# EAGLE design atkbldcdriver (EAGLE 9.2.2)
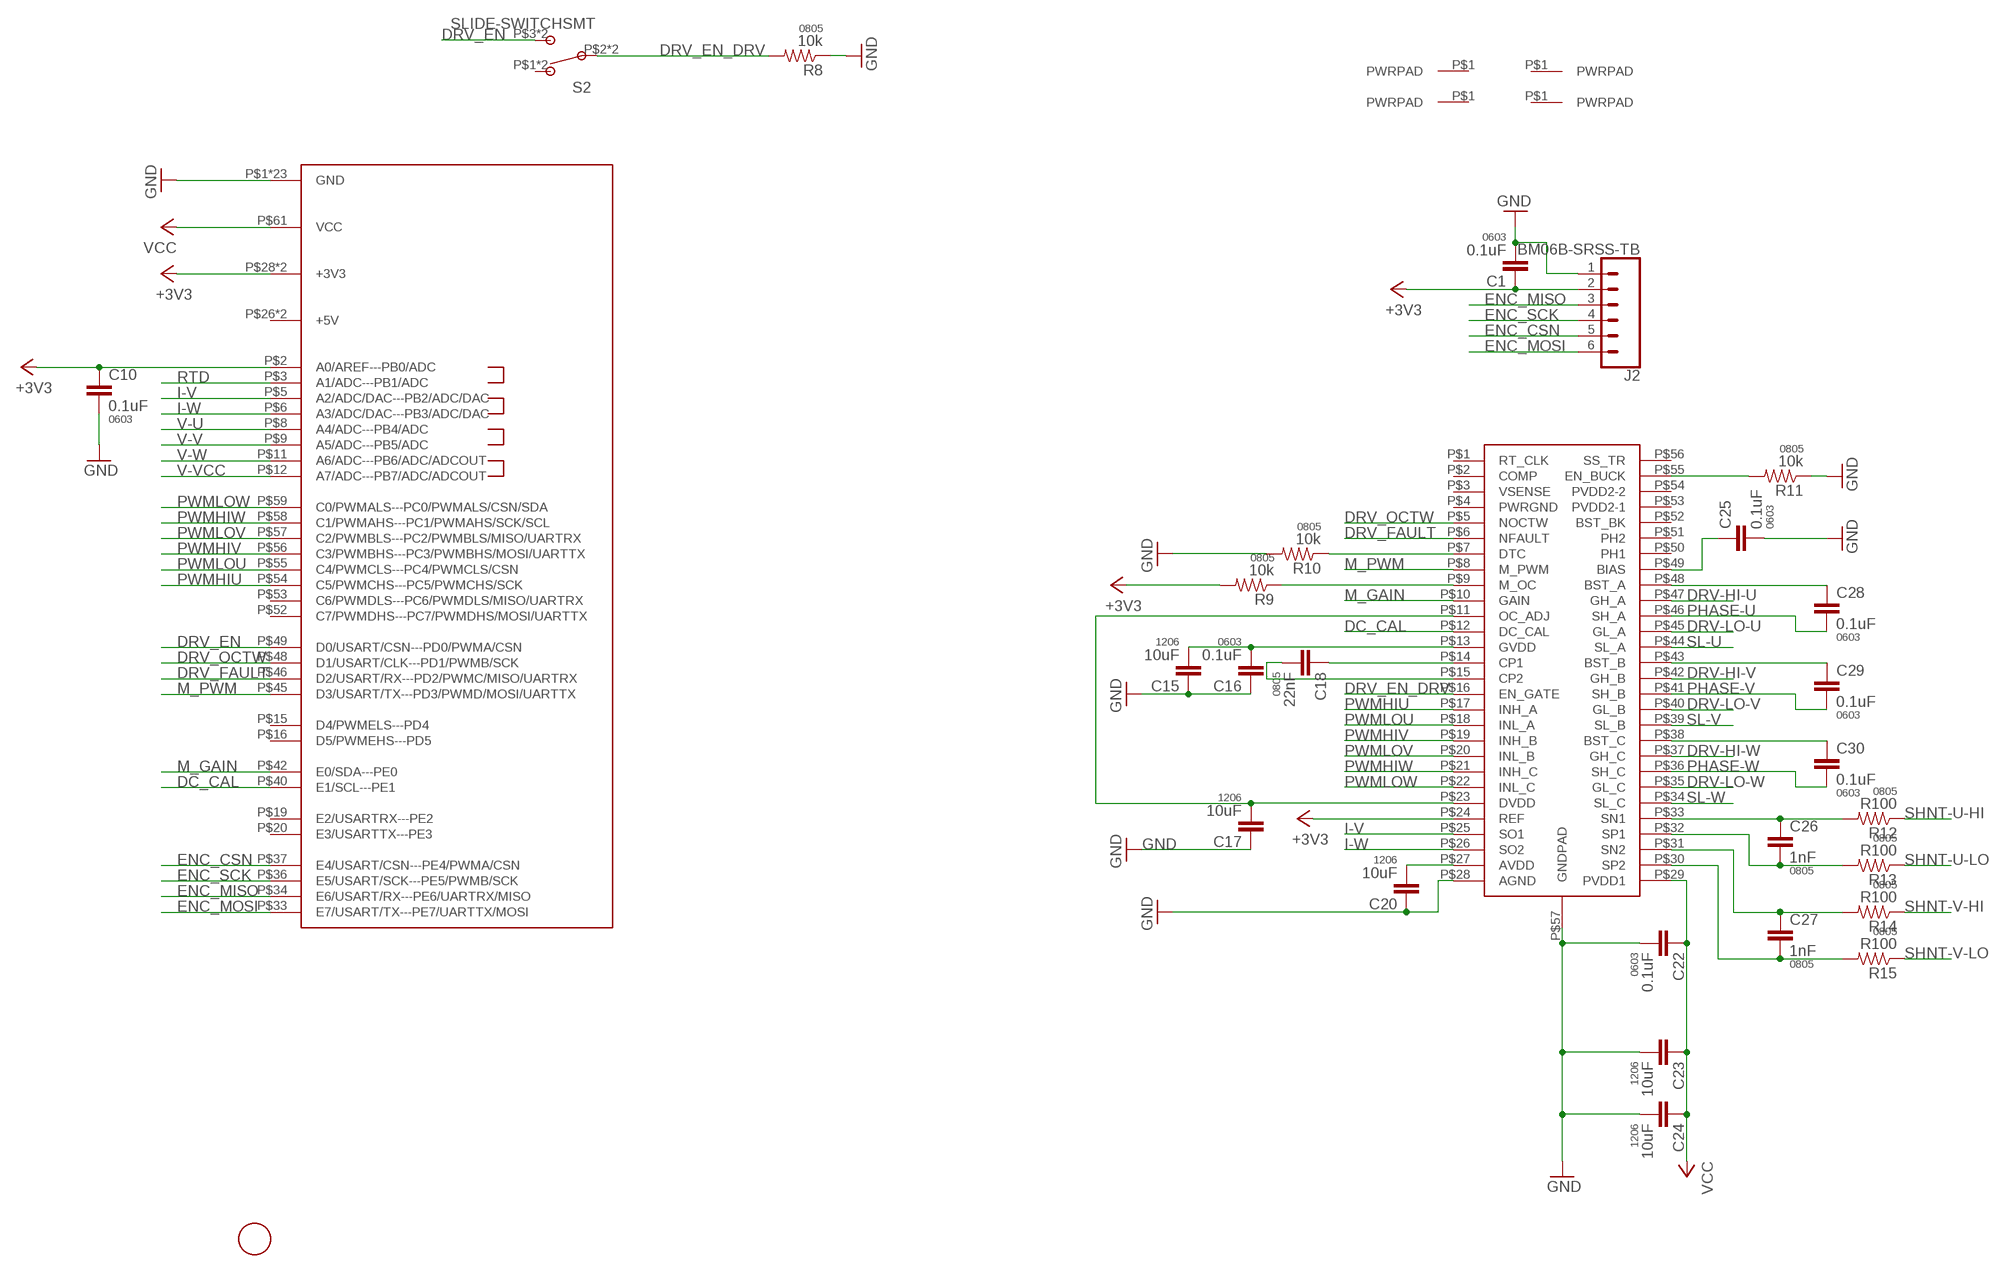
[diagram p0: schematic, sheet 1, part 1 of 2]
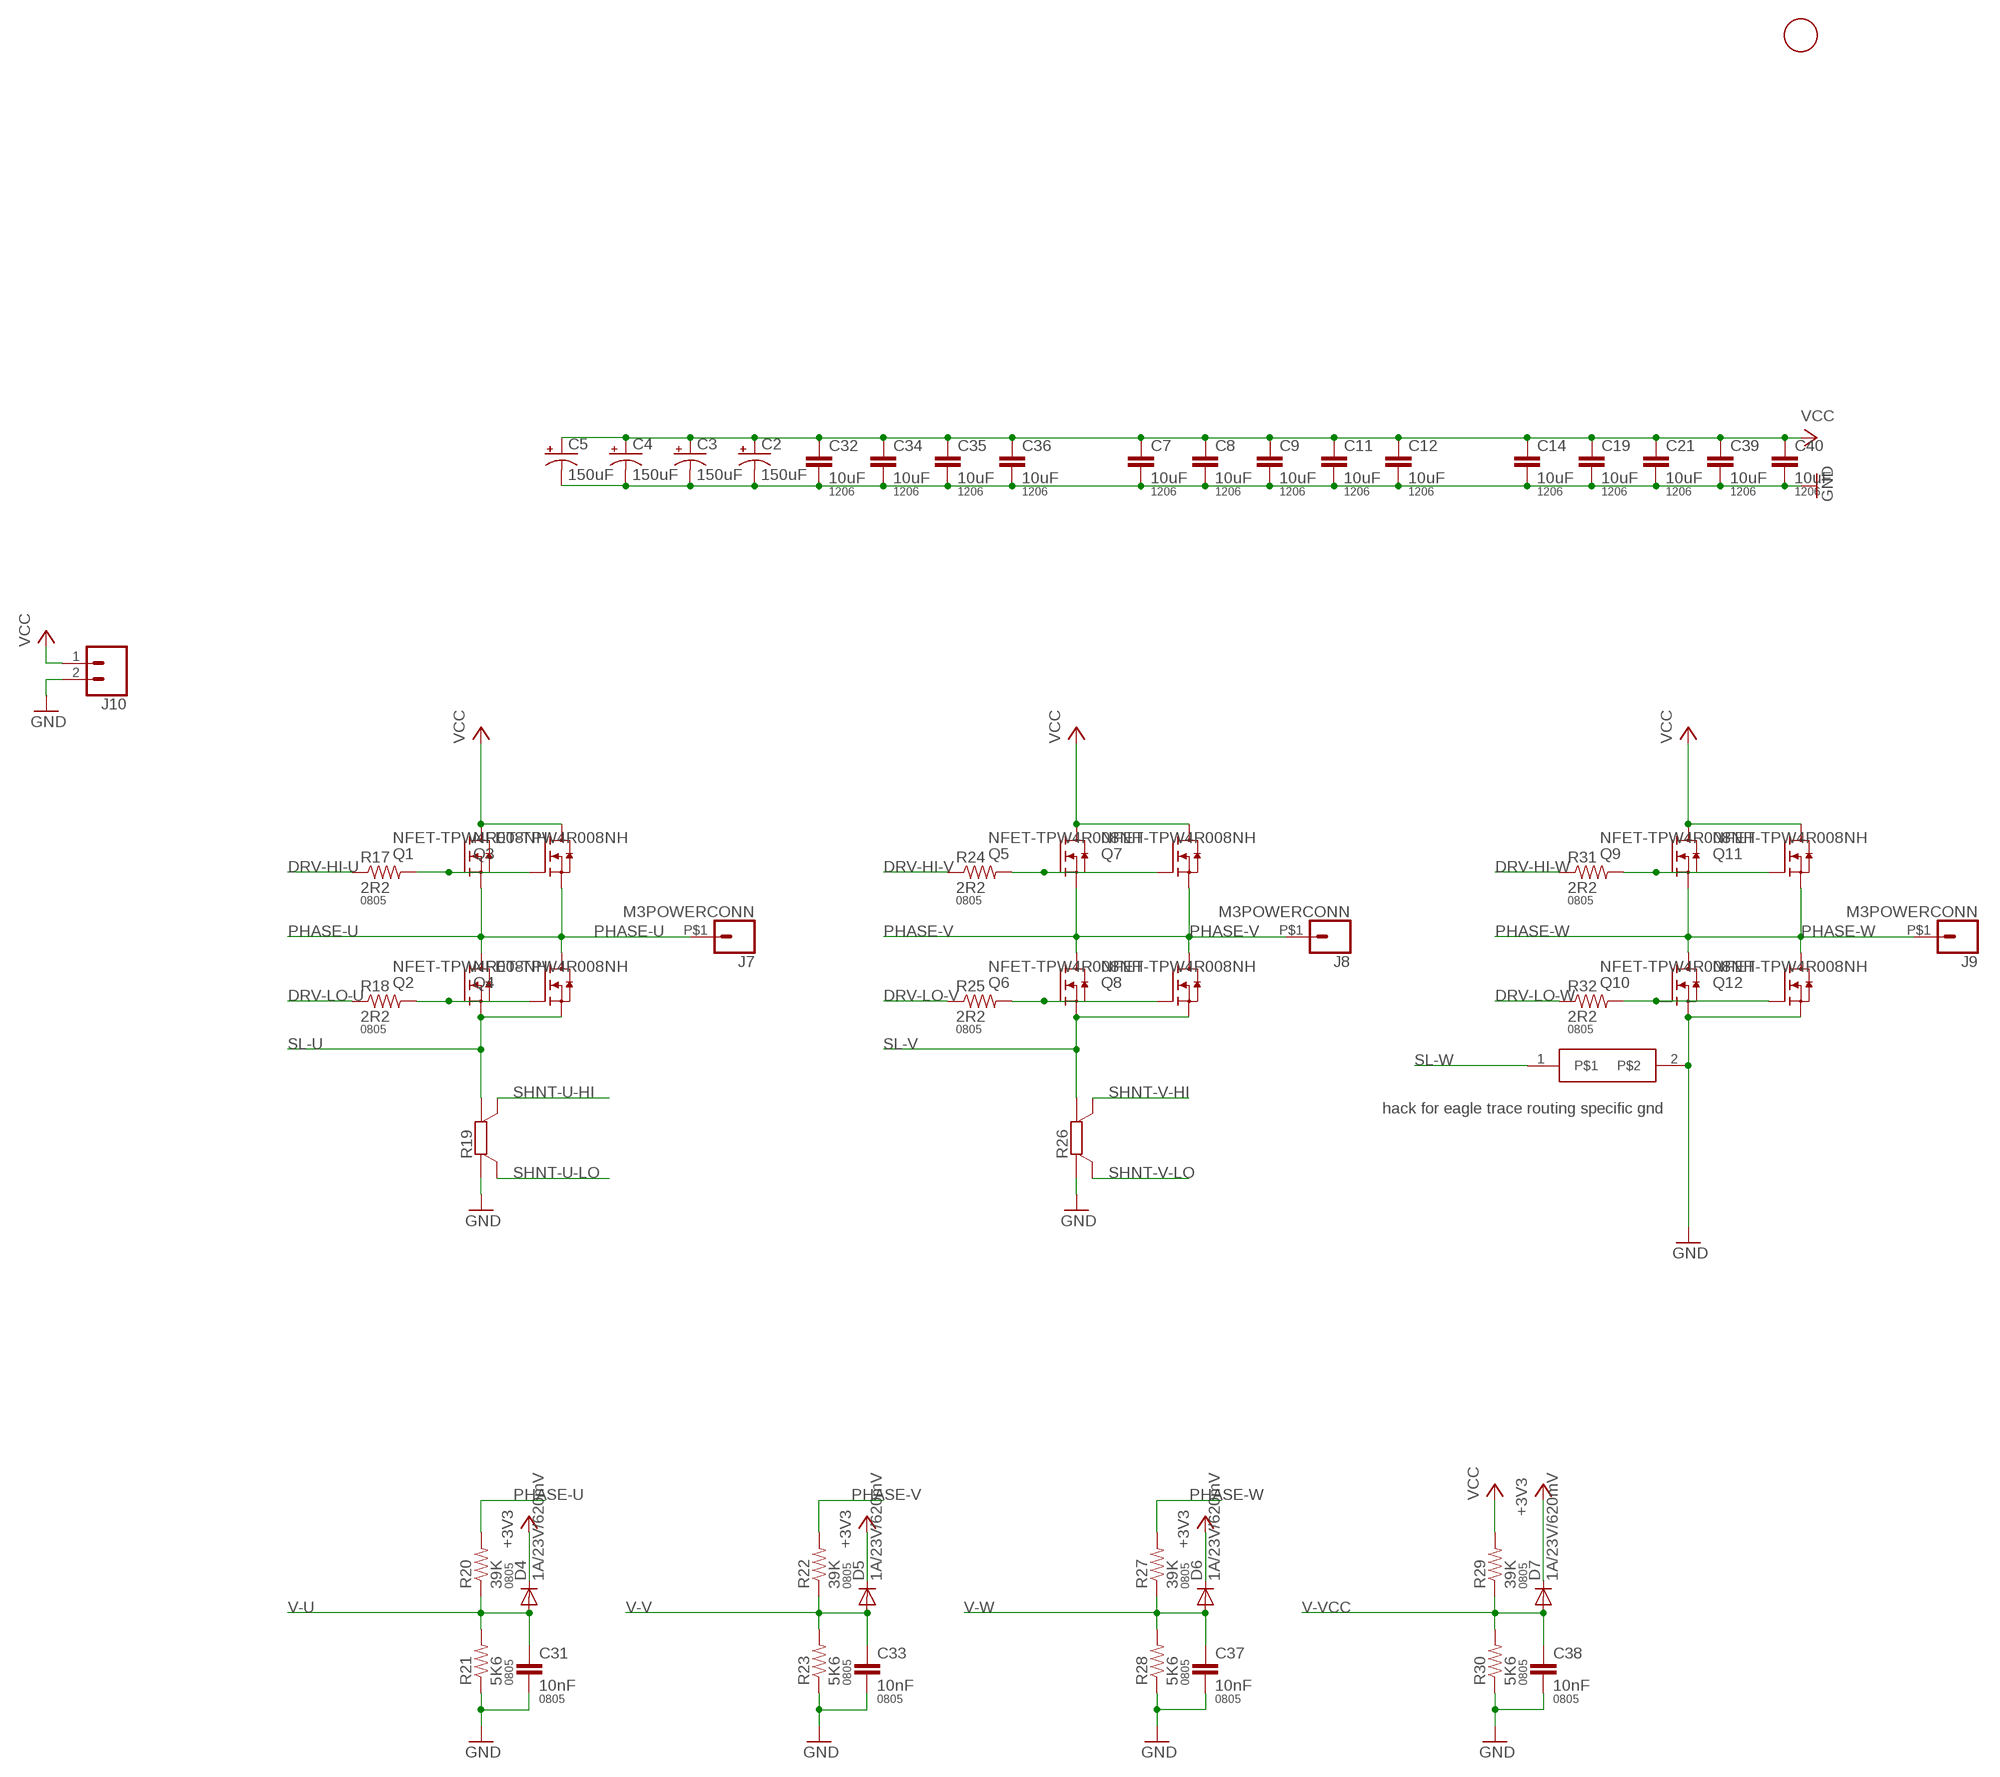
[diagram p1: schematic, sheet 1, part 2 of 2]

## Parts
C1  0.1uF  CAP0603-CAP  [0603-CAP]
C2  150uF  CAP-POL-6.6X6.6  [6.6X6.6-CAP]
C3  150uF  CAP-POL-6.6X6.6  [6.6X6.6-CAP]
C4  150uF  CAP-POL-6.6X6.6  [6.6X6.6-CAP]
C5  150uF  CAP-POL-6.6X6.6  [6.6X6.6-CAP]
C7  10uF  CAP1206  [1206]
C8  10uF  CAP1206  [1206]
C9  10uF  CAP1206  [1206]
C10  0.1uF  CAP0603-CAP  [0603-CAP]
C11  10uF  CAP1206  [1206]
C12  10uF  CAP1206  [1206]
C14  10uF  CAP1206  [1206]
C15  10uF  CAP1206  [1206]
C16  0.1uF  CAP0603-CAP  [0603-CAP]
C17  10uF  CAP1206  [1206]
C18  22nF  CAP0805  [0805]
C19  10uF  CAP1206  [1206]
C20  10uF  CAP1206  [1206]
C21  10uF  CAP1206  [1206]
C22  0.1uF  CAP0603-CAP  [0603-CAP]
C23  10uF  CAP1206  [1206]
C24  10uF  CAP1206  [1206]
C25  0.1uF  CAP0603-CAP  [0603-CAP]
C26  1nF  CAP0805  [0805]
C27  1nF  CAP0805  [0805]
C28  0.1uF  CAP0603-CAP  [0603-CAP]
C29  0.1uF  CAP0603-CAP  [0603-CAP]
C30  0.1uF  CAP0603-CAP  [0603-CAP]
C31  10nF  CAP0805  [0805]
C32  10uF  CAP1206  [1206]
C33  10nF  CAP0805  [0805]
C34  10uF  CAP1206  [1206]
C35  10uF  CAP1206  [1206]
C36  10uF  CAP1206  [1206]
C37  10nF  CAP0805  [0805]
C38  10nF  CAP0805  [0805]
C39  10uF  CAP1206  [1206]
C40  10uF  CAP1206  [1206]
D4  1A/23V/620mV  DIODEDIODE  [0805-DIODE]
D5  1A/23V/620mV  DIODEDIODE  [0805-DIODE]
D6  1A/23V/620mV  DIODEDIODE  [0805-DIODE]
D7  1A/23V/620mV  DIODEDIODE  [0805-DIODE]
J1  FIDUCIALRCT  [FIDUCIAL_RECT_1MM]
J2  BM06B-SRSS-TB  JST_6_PIN_HORIZONTAL  [JST-6-SMD-HORI-1.0MM]
J3  PWRPADM3  [PWRPAD_3-25MM]
J4  PWRPADM3  [PWRPAD_3-25MM]
J5  PWRPADM3  [PWRPAD_3-25MM]
J6  PWRPADM3  [PWRPAD_3-25MM]
J7  M3POWERCONN  [M3POWERCONN]
J8  M3POWERCONN  [M3POWERCONN]
J9  M3POWERCONN  [M3POWERCONN]
J10  CONN_021X02_NO_SILK  [1X02_NO_SILK]
J21  SL-LINK  [SL-LINK]
J22  FIDUCIALRCT  [FIDUCIAL_RECT_1MM]
J24  ATK-BFPPFX8-DAUGHTER  [ATK-BFPP-TOP-FX8-60]
Q1  NFET-TPW4R008NH  [DSOP-ADVANCE]
Q2  NFET-TPW4R008NH  [DSOP-ADVANCE]
Q3  NFET-TPW4R008NH  [DSOP-ADVANCE]
Q4  NFET-TPW4R008NH  [DSOP-ADVANCE]
Q5  NFET-TPW4R008NH  [DSOP-ADVANCE]
Q6  NFET-TPW4R008NH  [DSOP-ADVANCE]
Q7  NFET-TPW4R008NH  [DSOP-ADVANCE]
Q8  NFET-TPW4R008NH  [DSOP-ADVANCE]
Q9  NFET-TPW4R008NH  [DSOP-ADVANCE]
Q10  NFET-TPW4R008NH  [DSOP-ADVANCE]
Q11  NFET-TPW4R008NH  [DSOP-ADVANCE]
Q12  NFET-TPW4R008NH  [DSOP-ADVANCE]
R8  10k  RESISTOR0805-RES  [0805]
R9  10k  RESISTOR0805-RES  [0805]
R10  10k  RESISTOR0805-RES  [0805]
R11  10k  RESISTOR0805-RES  [0805]
R12  R100  RESISTOR0805-RES  [0805]
R13  R100  RESISTOR0805-RES  [0805]
R14  R100  RESISTOR0805-RES  [0805]
R15  R100  RESISTOR0805-RES  [0805]
R17  2R2  RESISTOR0805-RES  [0805]
R18  2R2  RESISTOR0805-RES  [0805]
R19  R_SHUNT2512  [R2512]
R20  39K  RESISTOR0805-RES  [0805]
R21  5K6  RESISTOR0805-RES  [0805]
R22  39K  RESISTOR0805-RES  [0805]
R23  5K6  RESISTOR0805-RES  [0805]
R24  2R2  RESISTOR0805-RES  [0805]
R25  2R2  RESISTOR0805-RES  [0805]
R26  R_SHUNT2512  [R2512]
R27  39K  RESISTOR0805-RES  [0805]
R28  5K6  RESISTOR0805-RES  [0805]
R29  39K  RESISTOR0805-RES  [0805]
R30  5K6  RESISTOR0805-RES  [0805]
R31  2R2  RESISTOR0805-RES  [0805]
R32  2R2  RESISTOR0805-RES  [0805]
S2  SLIDE-SWITCHSMT  [SLIDESWITCH-CL-SB-22A]
U5  DRV8302  [HTSSOP-56]

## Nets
+3V3: C1.1 C10.1 D4.2(C) D5.2(C) D6.2(C) D7.2(C) J2.2 J24.P$2(A0/AREF---PB0/ADC) J24.P$28(+3V3) J24.P$29(+3V3) R9.2 U5.P$24(REF)
CP1: C18.1 U5.P$14(CP1)
CP2: C18.2 U5.P$15(CP2)
DC_CAL: J24.P$40(E1/SCL---PE1) U5.P$12(DC_CAL)
DRV-HI-U: R17.1 U5.P$47(GH_A)
DRV-HI-V: R24.1 U5.P$42(GH_B)
DRV-HI-W: R31.1 U5.P$37(GH_C)
DRV-LO-U: R18.1 U5.P$45(GL_A)
DRV-LO-V: R25.1 U5.P$40(GL_B)
DRV-LO-W: R32.1 U5.P$35(GL_C)
DRV_EN: J24.P$49(D0/USART/CSN---PD0/PWMA/CSN) S2.P$3 S2.P$6
DRV_EN_DRV: R8.2 S2.P$2 S2.P$5 U5.P$16(EN_GATE)
DRV_FAULT: J24.P$46(D2/USART/RX---PD2/PWMC/MISO/UARTRX) U5.P$6(NFAULT)
DRV_OCTW: J24.P$48(D1/USART/CLK---PD1/PWMB/SCK) U5.P$5(NOCTW)
ENC_CSN: J2.5 J24.P$37(E4/USART/CSN---PE4/PWMA/CSN)
ENC_MISO: J2.3 J24.P$34(E6/USART/RX---PE6/UARTRX/MISO)
ENC_MOSI: J2.6 J24.P$33(E7/USART/TX---PE7/UARTTX/MOSI)
ENC_SCK: J2.4 J24.P$36(E5/USART/SCK---PE5/PWMB/SCK)
GND: C1.2 C2.- C3.- C4.- C5.- C7.2 C8.2 C9.2 C10.2 C11.2 C12.2 C14.2 C15.1 C16.1 C17.1 C19.2 C20.1 C21.2 C22.2 C23.2 C24.2 C25.2 C31.2 C32.2 C33.2 C34.2 C35.2 C36.2 C37.2 C38.2 C39.2 C40.2 J2.1 J10.2 J21.2 J24.P$1(GND) J24.P$4(GND) J24.P$7(GND) J24.P$10(GND) J24.P$13(GND) J24.P$14(GND) J24.P$17(GND) J24.P$18(GND) J24.P$21(GND) J24.P$30(GND) J24.P$31(GND) J24.P$32(GND) J24.P$35(GND) J24.P$38(GND) J24.P$39(GND) J24.P$41(GND) J24.P$43(GND) J24.P$44(GND) J24.P$47(GND) J24.P$50(GND) J24.P$51(GND) J24.P$60(GND) J24.P$62(GND) Q10.P$1(S) Q10.P$2(S) Q10.P$3(S) Q12.P$1(S) Q12.P$2(S) Q12.P$3(S) R8.1 R10.2 R11.1 R19.B R21.1 R23.1 R26.B R28.1 R30.1 U5.P$28(AGND) U5.P$57(GNDPAD)
I-V: J24.P$5(A2/ADC/DAC---PB2/ADC/DAC) U5.P$25(SO1)
I-W: J24.P$6(A3/ADC/DAC---PB3/ADC/DAC) U5.P$26(SO2)
M_GAIN: J24.P$42(E0/SDA---PE0) U5.P$10(GAIN)
M_PWM: J24.P$45(D3/USART/TX---PD3/PWMD/MOSI/UARTTX) U5.P$8(M_PWM)
N$2: Q2.P$4(G) Q4.P$4(G) R18.2
N$3: Q1.P$4(G) Q3.P$4(G) R17.2
N$4: Q5.P$4(G) Q7.P$4(G) R24.2
N$5: Q9.P$4(G) Q11.P$4(G) R31.2
N$6: Q10.P$4(G) Q12.P$4(G) R32.2
N$7: C30.1 U5.P$38(BST_C)
N$8: C29.1 U5.P$43(BST_B)
N$9: C28.1 U5.P$48(BST_A)
N$10: R11.2 U5.P$55(EN_BUCK)
N$11: C20.2 U5.P$27(AVDD)
N$13: C26.1 R12.2 U5.P$33(SN1)
N$14: C26.2 R13.2 U5.P$32(SP1)
N$15: C27.1 R14.2 U5.P$31(SN2)
N$16: C27.2 R15.2 U5.P$30(SP2)
N$18: C15.2 C16.2 U5.P$13(GVDD)
N$19: C25.1 U5.P$49(BIAS)
N$20: C17.2 U5.P$11(OC_ADJ) U5.P$23(DVDD)
N$21: R10.1 U5.P$7(DTC)
N$24: Q6.P$4(G) Q8.P$4(G) R25.2
N$25: R9.1 U5.P$9(M_OC)
PHASE-U: C28.2 J7.P$1 Q1.P$1(S) Q1.P$2(S) Q1.P$3(S) Q2.P$5(D) Q3.P$1(S) Q3.P$2(S) Q3.P$3(S) Q4.P$5(D) R20.2 U5.P$46(SH_A)
PHASE-V: C29.2 J8.P$1 Q5.P$1(S) Q5.P$2(S) Q5.P$3(S) Q6.P$5(D) Q7.P$1(S) Q7.P$2(S) Q7.P$3(S) Q8.P$5(D) R22.2 U5.P$41(SH_B)
PHASE-W: C30.2 J9.P$1 Q9.P$1(S) Q9.P$2(S) Q9.P$3(S) Q10.P$5(D) Q11.P$1(S) Q11.P$2(S) Q11.P$3(S) Q12.P$5(D) R27.2 U5.P$36(SH_C)
PWMHIU: J24.P$54(C5/PWMCHS---PC5/PWMCHS/SCK) U5.P$17(INH_A)
PWMHIV: J24.P$56(C3/PWMBHS---PC3/PWMBHS/MOSI/UARTTX) U5.P$19(INH_B)
PWMHIW: J24.P$58(C1/PWMAHS---PC1/PWMAHS/SCK/SCL) U5.P$21(INH_C)
PWMLOU: J24.P$55(C4/PWMCLS---PC4/PWMCLS/CSN) U5.P$18(INL_A)
PWMLOV: J24.P$57(C2/PWMBLS---PC2/PWMBLS/MISO/UARTRX) U5.P$20(INL_B)
PWMLOW: J24.P$59(C0/PWMALS---PC0/PWMALS/CSN/SDA) U5.P$22(INL_C)
RTD: J24.P$3(A1/ADC---PB1/ADC)
SHNT-U-HI: R12.1 R19.SA
SHNT-U-LO: R13.1 R19.SB
SHNT-V-HI: R14.1 R26.SA
SHNT-V-LO: R15.1 R26.SB
SL-U: Q2.P$1(S) Q2.P$2(S) Q2.P$3(S) Q4.P$1(S) Q4.P$2(S) Q4.P$3(S) R19.A U5.P$44(SL_A)
SL-V: Q6.P$1(S) Q6.P$2(S) Q6.P$3(S) Q8.P$1(S) Q8.P$2(S) Q8.P$3(S) R26.A U5.P$39(SL_B)
SL-W: J21.1 U5.P$34(SL_C)
V-U: C31.1 D4.1(A) J24.P$8(A4/ADC---PB4/ADC) R20.1 R21.2
V-V: C33.1 D5.1(A) J24.P$9(A5/ADC---PB5/ADC) R22.1 R23.2
V-VCC: C38.1 D7.1(A) J24.P$12(A7/ADC---PB7/ADC/ADCOUT) R29.1 R30.2
V-W: C37.1 D6.1(A) J24.P$11(A6/ADC---PB6/ADC/ADCOUT) R27.1 R28.2
VCC: C2.+ C3.+ C4.+ C5.+ C7.1 C8.1 C9.1 C11.1 C12.1 C14.1 C19.1 C21.1 C22.1 C23.1 C24.1 C32.1 C34.1 C35.1 C36.1 C39.1 C40.1 J10.1 J24.P$61(VCC) Q1.P$5(D) Q3.P$5(D) Q5.P$5(D) Q7.P$5(D) Q9.P$5(D) Q11.P$5(D) R29.2 U5.P$29(PVDD1)
Unconnected: J3.P$1(PWRPAD) J4.P$1(PWRPAD) J5.P$1(PWRPAD) J6.P$1(PWRPAD) J24.P$15(D4/PWMELS---PD4) J24.P$16(D5/PWMEHS---PD5) J24.P$19(E2/USARTRX---PE2) J24.P$20(E3/USARTTX---PE3) J24.P$26(+5V) J24.P$27(+5V) J24.P$52(C7/PWMDHS---PC7/PWMDHS/MOSI/UARTTX) J24.P$53(C6/PWMDLS---PC6/PWMDLS/MISO/UARTRX) S2.P$1 S2.P$4 U5.P$1(RT_CLK) U5.P$2(COMP) U5.P$3(VSENSE) U5.P$4(PWRGND) U5.P$50(PH1) U5.P$51(PH2) U5.P$52(BST_BK) U5.P$53(PVDD2-1) U5.P$54(PVDD2-2) U5.P$56(SS_TR)

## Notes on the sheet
- hack for eagle trace routing specific gnd

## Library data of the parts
C1 C10 C16 C22 C25 C28-C30 = borkedlabs-passives:CAP: Capacitor; PACKAGE: 0603
C2-C5 = borkedlabs-passives:CAP-POL
C7-C9 C11 C12 C14 C15 C17 C19-C21 C23 C24 C32 C34-C36 C39 C40 = borkedlabs-passives:CAP: Capacitor; PACKAGE: 1206
C18 C26 C27 C31 C33 C37 C38 = borkedlabs-passives:CAP: Capacitor; PACKAGE: 0805
D4-D7 = passives:DIODE: DIODE
J1 J22 = connector:FIDUCIAL: For use by pick and place machines to calibrate the vision/machine, 1mm
J2 = connector:JST_6_PIN_HORIZONTAL: JST 6 pin horizontal connector JST-SH type. Here is the connector we sell at SparkFun: name (XXX-00000) Datasheet It was used on these SparkFun products: name (XXX-00000) name (XXX-00000); PROD_ID: XXX-00000
J3-J6 = power:PWRPAD
J7-J9 = connector:M3POWERCONN
J10 = SparkFun-Connectors:CONN_02: Multi connection point. Often used as Generic Header-pin footprint for 0.1 inch spaced/style header connections
J21 = power:SL-LINK
J24 = connector:ATK-BFPP
Q1-Q12 = power:NFET-TPW4R008NH
R8-R15 R17 R18 R20-R25 R27-R32 = borkedlabs-passives:RESISTOR: Resistor; PACKAGE: 0805
R19 R26 = power:R_SHUNT: Resistor Basic schematic elements and footprints for 0603, 1206, and PTH resistors.
S2 = fab:SLIDE-SWITCH: SMD slide-switch AYZ0102AGRLC as found in the fablab inventory. Includes the mounting holes. Made by Zaerc.
U5 = power:DRV8302

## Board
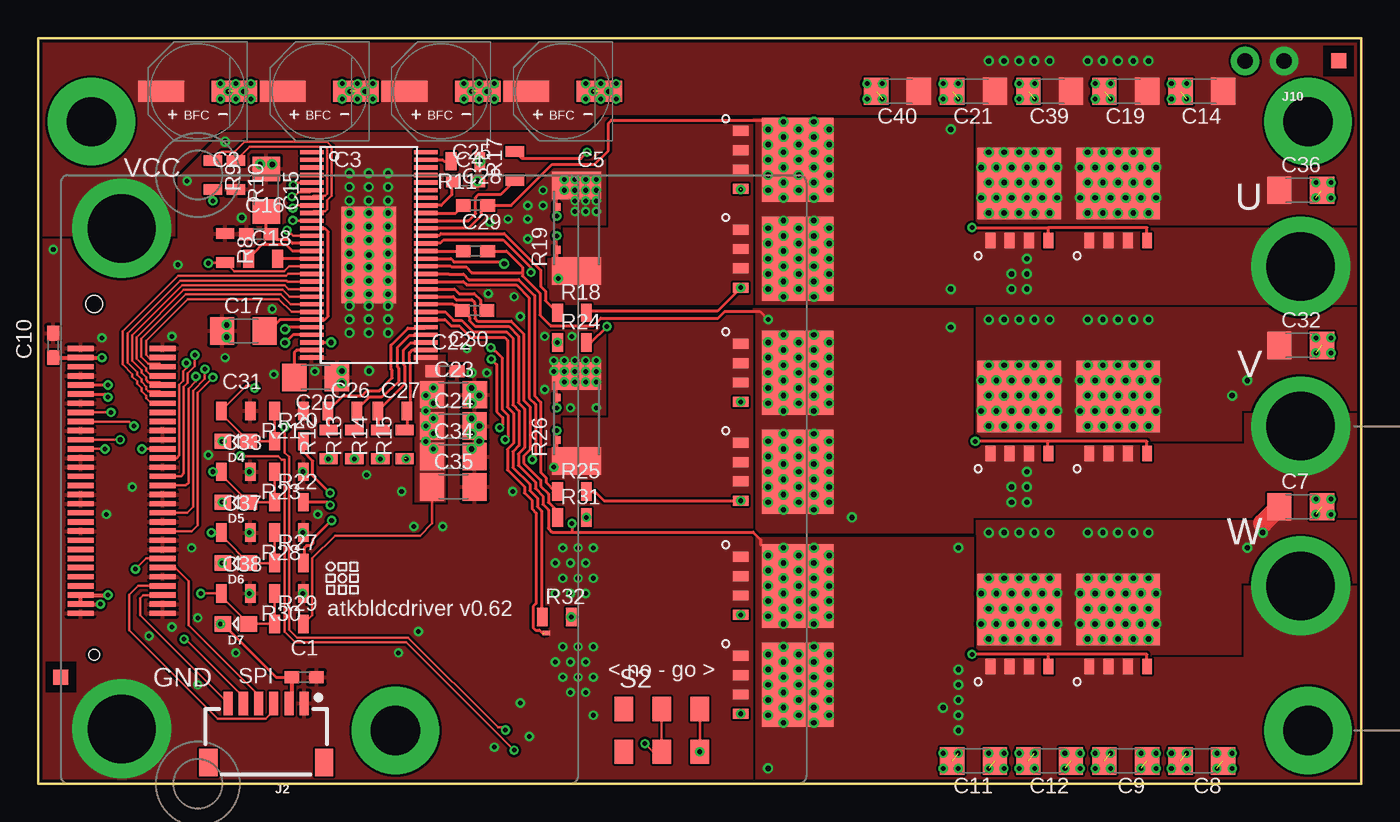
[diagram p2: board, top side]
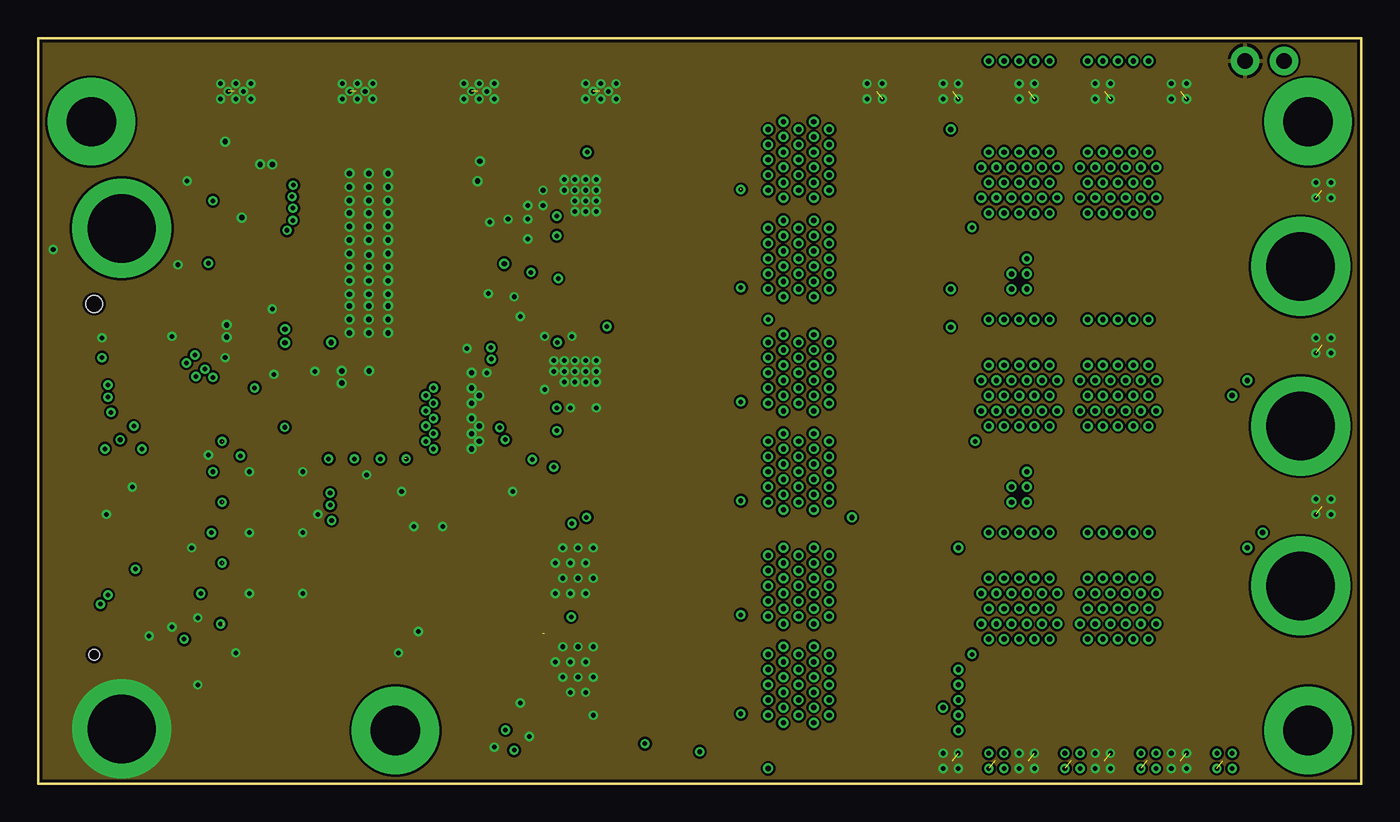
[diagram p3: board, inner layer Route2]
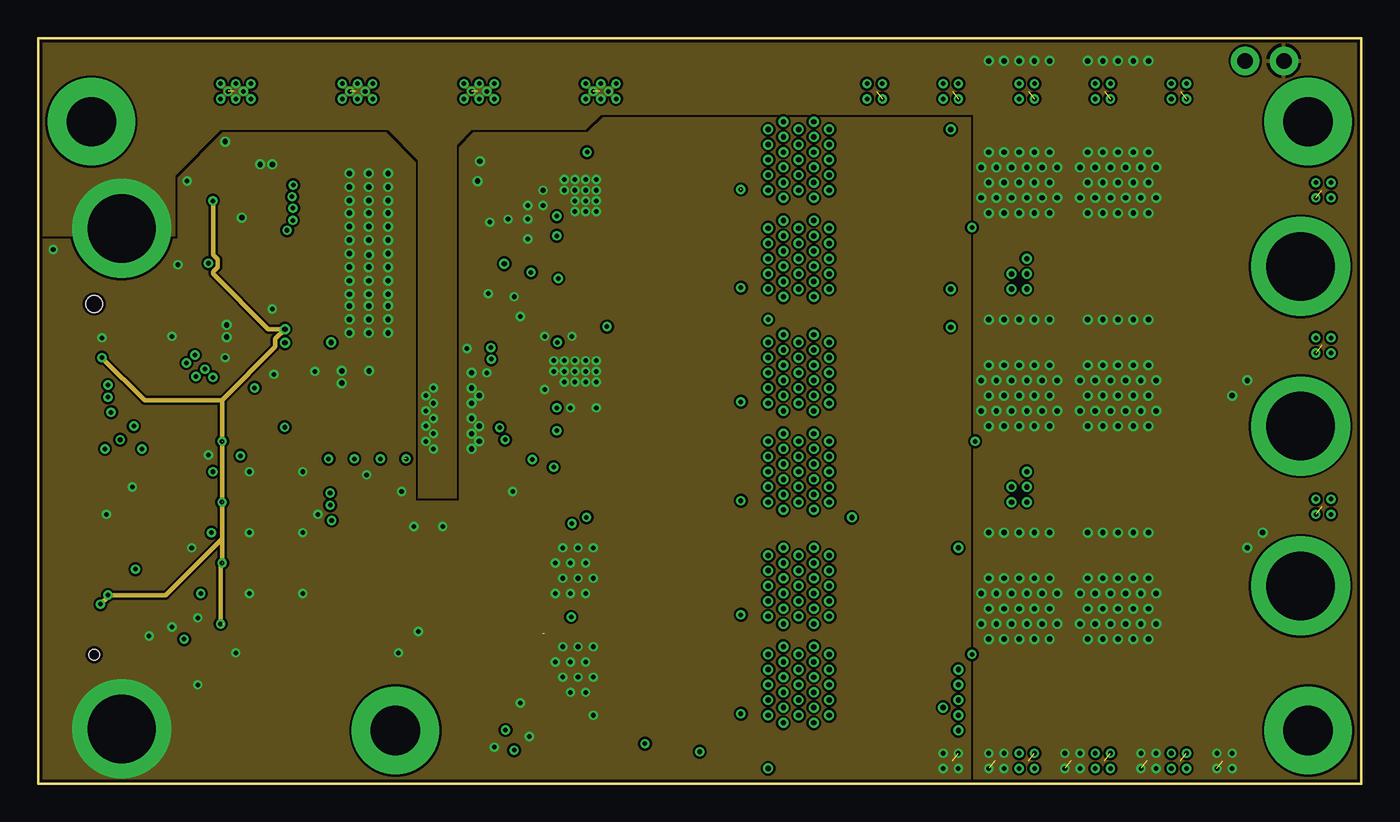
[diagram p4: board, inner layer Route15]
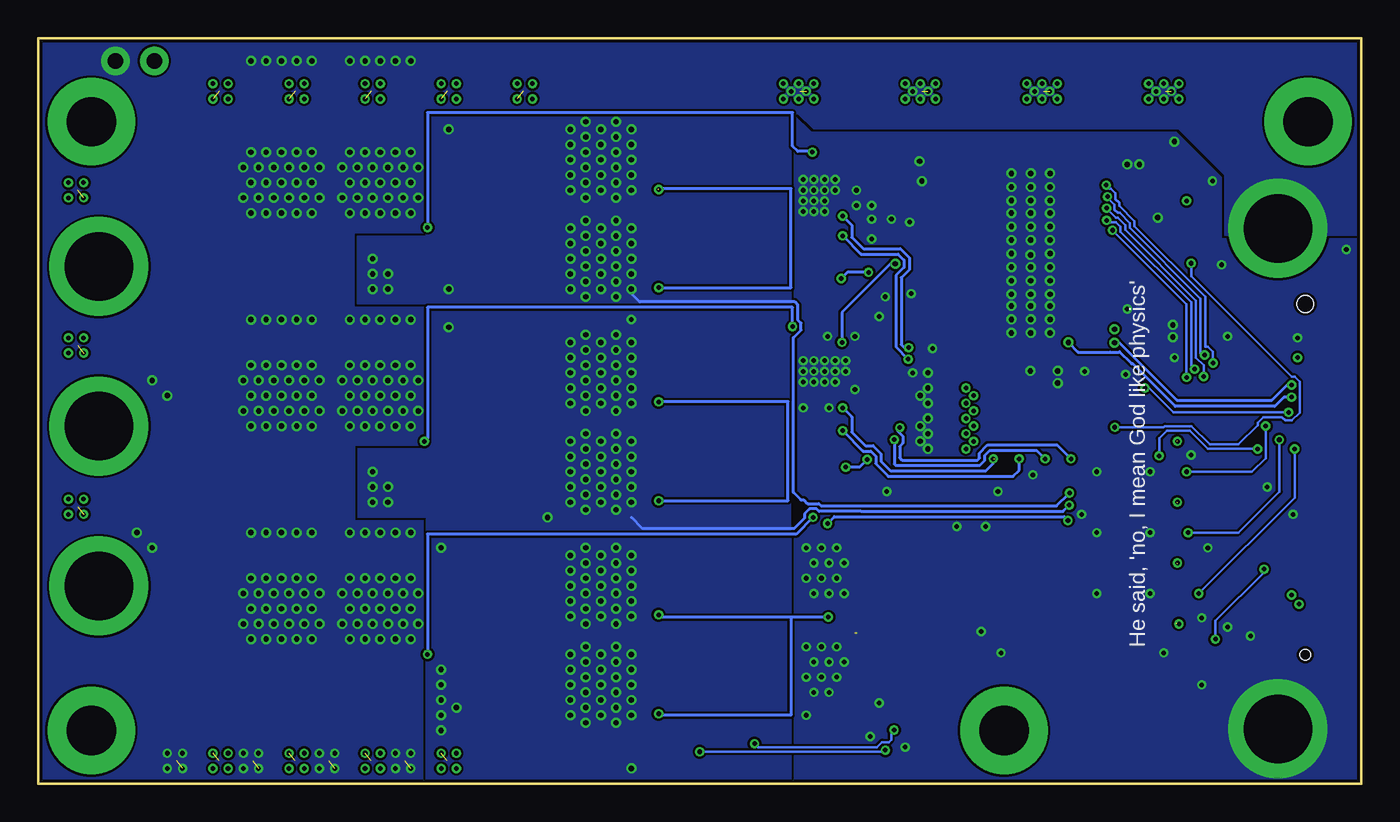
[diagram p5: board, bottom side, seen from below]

Size 87 x 49 mm. Coordinates in mm from the lower left corner, seen from the top.
Outline: 0,49 0,0 87,0 87,49 0,49
Copper layers (1+2*15+16): Top 0.035mm / dielectric 1.5mm / Route2 0.035mm / dielectric 0.15mm / Route15 0.035mm / dielectric 0.2mm / Bottom 0.035mm
Design rules "default *": minimum track width 6mil, minimum drill 0.3mm, track to track 6mil, track to pad 6mil, pad to pad 6mil, via to via 6mil, smd to smd 6mil, copper to edge 8mil, drill to drill 8mil, minimum pad ring 10mil, minimum via ring 6mil, stop-mask expansion 4mil, vias tented up to drill 20mil, thermal gap 8mil

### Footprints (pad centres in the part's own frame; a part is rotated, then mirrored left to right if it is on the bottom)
0603-CAP = smd 0.96 x 0.8: 1 -0.8,0; 2 0.8,0
6.6X6.6-CAP = smd 3 x 1.4: + 2.4,0; - -2.4,0
1206 = smd 1.6 x 1.8: 1 -1.4,0; 2 1.4,0
0805 = smd 0.7 x 1.2: 1 -0.95,0; 2 0.95,0
0805-DIODE = smd 1.1 x 1: 1 -0.85,0; 2 0.85,0
FIDUCIAL_RECT_1MM = smd 1 x 1: P$1 0,0
JST-6-SMD-HORI-1.0MM = smd 0.6 x 1.55: 1 -2.5,-4.775; 2 -1.5,-4.775; 3 -0.5,-4.775; 4 0.5,-4.775; 5 1.5,-4.775; 6 2.5,-4.775 | smd 1.2 x 1.8: M1 -3.8,-0.9; M2 3.8,-0.9
PWRPAD_3-25MM = drill 3.25 pad 5.75: P$1 0,0
M3POWERCONN = drill 4.5 pad 6.5: P$1 0,0
1X02_NO_SILK = drill 1.016 pad 1.88: 1 0,0; 2 2.54,0
SL-LINK = smd 0.3 x 0.3: 1 -0.1,0; 2 0.1,0
ATK-BFPP-TOP-FX8-60 = smd 0.35 x 1.7: P$1 -8.6,-2.7; P$2 -8,-2.7; P$3 -7.4,-2.7; P$4 -6.8,-2.7; P$5 -6.2,-2.7; P$6 -5.6,-2.7; P$7 -5,-2.7; P$8 -4.4,-2.7; P$9 -3.8,-2.7; P$10 -3.2,-2.7; P$11 -2.6,-2.7; P$12 -2,-2.7; P$13 -1.4,-2.7; P$14 -0.8,-2.7; P$15 -0.2,-2.7; P$16 0.4,-2.7; P$17 1,-2.7; P$18 1.6,-2.7; P$19 2.2,-2.7; P$20 2.8,-2.7; P$21 3.4,-2.7; P$22 4,-2.7; P$23 4.6,-2.7; P$24 5.2,-2.7; P$25 5.8,-2.7; P$26 6.4,-2.7; P$27 7,-2.7; P$28 7.6,-2.7; P$29 8.2,-2.7; P$30 8.8,-2.7; P$31 8.8,2.7; P$32 8.2,2.7; P$33 7.6,2.7; P$34 7,2.7; P$35 6.4,2.7; P$36 5.8,2.7; P$37 5.2,2.7; P$38 4.6,2.7; P$39 4,2.7; P$40 3.4,2.7; P$41 2.8,2.7; P$42 2.2,2.7; P$43 1.6,2.7; P$44 1,2.7; P$45 0.4,2.7; P$46 -0.2,2.7; P$47 -0.8,2.7; P$48 -1.4,2.7; P$49 -2,2.7; P$50 -2.6,2.7; P$51 -3.2,2.7; P$52 -3.8,2.7; P$53 -4.4,2.7; P$54 -5,2.7; P$55 -5.6,2.7; P$56 -6.2,2.7; P$57 -6.8,2.7; P$58 -7.4,2.7; P$59 -8,2.7; P$60 -8.6,2.7 | drill 4.5 pad 6.5: P$61 -16.5,0; P$62 16.4,0 | hole 1.1: -11.525,-1.8 | hole 0.7: 11.525,-1.8
DSOP-ADVANCE = smd 0.65 x 1: P$1 -1.905,-2.8; P$2 -0.635,-2.8; P$3 0.635,-2.8; P$4 1.905,-2.8 | smd 5.5 x 4.7: P$5 0,0.95
R2512 = smd 1.8 x 3.2: A -2.8,0; B 2.8,0 | smd 0.5 x 0.5: SA -1.414,1.3; SB 1.386,1.3
SLIDESWITCH-CL-SB-22A = smd 1.2 x 1.6: P$1 -2.5,1.4; P$2 0,1.4; P$3 2.5,1.4; P$4 -2.5,-1.4; P$5 0,-1.4; P$6 2.5,-1.4
HTSSOP-56 = smd 1.549 x 0.279: P$1 -3.75,6.75; P$2 -3.75,6.25; P$3 -3.75,5.75; P$4 -3.75,5.25; P$5 -3.75,4.75; P$6 -3.75,4.25; P$7 -3.75,3.75; P$8 -3.75,3.25; P$9 -3.75,2.75; P$10 -3.75,2.25; P$11 -3.75,1.75; P$12 -3.75,1.25; P$13 -3.75,0.75; P$14 -3.75,0.25; P$15 -3.75,-0.25; P$16 -3.75,-0.75; P$17 -3.75,-1.25; P$18 -3.75,-1.75; P$19 -3.75,-2.25; P$20 -3.75,-2.75; P$21 -3.75,-3.25; P$22 -3.75,-3.75; P$23 -3.75,-4.25; P$24 -3.75,-4.75; P$25 -3.75,-5.25; P$26 -3.75,-5.75; P$27 -3.75,-6.25; P$28 -3.75,-6.75; P$29 3.75,-6.75; P$30 3.75,-6.25; P$31 3.75,-5.75; P$32 3.75,-5.25; P$33 3.75,-4.75; P$34 3.75,-4.25; P$35 3.75,-3.75; P$36 3.75,-3.25; P$37 3.75,-2.75; P$38 3.75,-2.25; P$39 3.75,-1.75; P$40 3.75,-1.25; P$41 3.75,-0.75; P$42 3.75,-0.25; P$43 3.75,0.25; P$44 3.75,0.75; P$45 3.75,1.25; P$46 3.75,1.75; P$47 3.75,2.25; P$48 3.75,2.75; P$49 3.75,3.25; P$50 3.75,3.75; P$51 3.75,4.25; P$52 3.75,4.75; P$53 3.75,5.25; P$54 3.75,5.75; P$55 3.75,6.25; P$56 3.75,6.75 | smd 3.581 x 6.35: P$57 0,0

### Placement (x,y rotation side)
C1  17.5,7 0 top
C2  10.5,45.5 180 top
C3  18.5,45.5 180 top
C4  26.5,45.5 180 top
C5  34.5,45.5 180 top
C7  83,18.2 0 top
C8  76.5,1.5 180 top
C9  71.5,1.5 180 top
C10  1,28.8 90 top
C11  61.5,1.5 180 top
C12  66.5,1.5 180 top
C14  76.5,45.5 180 top
C15  15,39 270 top
C16  14.5,36.1 0 top
C17  13.5,29.75 0 top
C18  14.8,34.5 0 top
C19  71.5,45.5 180 top
C20  18.25,26.7 180 top
C21  61.5,45.5 180 top
C22  26.75,27.1 0 top
C23  27.31,25.56 0 top
C24  27.3,23.5 0 top
C25  28.1,39.6 0 top
C26  20,24.5 0 top
C27  23.3,24.5 0 top
C28  28.75,38 0 top
C29  28.75,35 0 top
C30  28.7,31.1 180 top
C31  13,24.5 0 top
C32  83,28.8 0 top
C33  13,20.5 0 top
C34  27.3,21.5 0 top
C35  27.3,19.5 0 top
C36  83,39 0 top
C37  13,16.5 0 top
C38  13,12.5 0 top
C39  66.5,45.5 180 top
C40  56.5,45.5 180 top
D4  13,22.5 180 top
D5  13,18.5 180 top
D6  13,14.5 180 top
D7  13,10.5 180 top
J1  85.5,47.5 0 top
J2  15,0.5 180 top
J3  23.5,3.5 0 top
J4  83.5,3.5 0 top
J5  83.5,43.5 0 top
J6  3.5,43.5 0 top
J7  83,34 0 top
J8  83,23.5 0 top
J9  83,13 0 top
J10  81.9,47.5 180 top
J21  33.4,9.9 0 top
J22  1.5,7 0 top
J24  5.5,20 270 top
Q1  64.5,38.5 0 top
Q2  49,34.5 270 top
Q3  71,38.5 0 top
Q4  49,41 270 top
Q5  71,24.5 0 top
Q6  49,27 270 top
Q7  64.5,24.5 0 top
Q8  49,20.5 270 top
Q9  64.5,10.5 0 top
Q10  49,6.5 270 top
Q11  71,10.5 0 top
Q12  49,13 270 top
R8  12.3,35.2 270 top
R9  11.5,40 270 top
R10  13,40 270 top
R11  28.1,40.9 180 top
R12  19.1,22.3 90 top
R13  20.8,22.3 90 top
R14  22.5,22.3 90 top
R15  24.1,22.3 90 top
R17  31.35,40.6 90 top
R18  35.1,30.95 0 top
R19  35.4,36.5 90 top
R20  16.5,22.5 0 top
R21  16.5,24.5 180 top
R22  16.5,18.5 0 top
R23  16.5,20.5 180 top
R24  35.1,29 0 top
R25  35.1,19.2 0 top
R26  35.4,24 90 top
R27  16.5,14.5 0 top
R28  16.5,16.5 180 top
R29  16.5,10.5 0 top
R30  16.5,12.5 180 top
R31  35.1,17.5 0 top
R32  34.1,10.95 0 top
S2  41,3.5 0 top
U5  21.75,34.75 0 top
U$2  [CBA-SILK-LOGO]  20,13.5 0 top

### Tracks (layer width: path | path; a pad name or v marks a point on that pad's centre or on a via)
+3V3  (via drill 0.3, 0.35)  (4 unrouted)
  Top 0.203: U5.P$24 16.36,30 v16.23,29.87 | D7.2 15.65,7 C1.1 | v11.5,38.3 R9.2
  Top 0.254: J2.2 16.7,5.47 C1.1 | v4.6,12.4 J24.P$28 J24.P$29 v4.1,11.8 | C10.1 J24.P$2 v4.2,28
  Route15 0.305: v4.1,11.8 4.6,12.3 v4.6,12.4 8.4,12.4 12.1,16.1 | 12.1,16.1 v12.1,14.5 12,14.4 v12,10.5 | 12.1,16.1 v12.1,18.5 12.1,20.24 12.11,20.25 12.11,20.75 12.1,20.76 v12.1,22.5 12.1,25.2 | 12.1,25.2 15.6,28.7 15.6,29.24 v16.23,29.87 15.13,29.87 11.5,33.5 11.5,33.64 11.81,33.95 11.81,34.45 11.5,34.76 v11.5,38.3 | v4.2,28 7,25.2 12.1,25.2
  Bottom 0.152: v12.1,14.5 12.2,14.4 | v12,10.5 12.2,10.5
CP1
  Top 0.203: U5.P$14 16.73,35 16.33,35.41 14.71,35.41 C18.1
CP2
  Top 0.203: U5.P$15 C18.2
DC_CAL  (via drill 0.3)
  Top 0.152: U5.P$12 16.77,36 16.63,36.14 16.6,36.14 v16.37,36.37 | v11.5,26.7 10.5,25.7 10.5,17 10.1,16.6 J24.P$40
  Bottom 0.152: v16.37,36.37 11.5,31.5 v11.5,26.7
DRV-HI-U
  Top 0.203: U5.P$47 28.3,37 28.77,37.47 28.77,38.53 28.94,38.7 30.41,38.7 R17.1
DRV-HI-V  (via drill 0.3, 0.35)
  Top 0.203: U5.P$42 27.14,34.5 27.34,34.3 30.52,34.3 v30.65,34.17
  Bottom 0.203: v30.65,34.17 30.95,34.17 34.15,30.97 R24.1
  other vias: 34.15,29
DRV-HI-W
  Top 0.203: U5.P$37 27.3,32 27.5,31.8 28.51,31.8 28.68,31.63 28.68,31.1 28.71,31.07 28.71,30.57 28.89,30.4 31.1,30.4 31.93,29.57 31.93,25.18 32.34,24.78 32.34,21.93 31.93,21.53 31.93,21.07 33.05,19.96 33.05,19.55 33.55,19.05 33.55,18.5 34.15,17.89 R31.1
DRV-LO-U
  Top 0.203: U5.P$45 25.55,36.05 26.4,36.05 26.5,36.15 30.65,36.15 33.05,33.75 33.05,32.68 33.36,32.37 33.36,31.74 R18.1
DRV-LO-V
  Top 0.203: U5.P$40 26.99,33.5 27.01,33.48 27.97,33.48 28.32,33.13 31.59,33.13 32.64,32.08 32.64,25.48 33.05,25.08 33.05,20.46 33.4,20.1 33.4,19.8 34,19.2 R25.1 34.15,19.59
DRV-LO-W
  Top 0.203: U5.P$35 | U5.P$35 26.76,31 27.32,30.45 27.84,30.45 28.59,29.69 30.8,29.69 31.22,29.27 31.22,24.89 31.62,24.49 31.62,22.23 31.22,21.82 31.22,20.77 32.34,19.66 32.34,19.26 32.84,18.76 32.84,18.2 33.1,17.93 33.1,11 R32.1
DRV_EN  (via drill 0.3)
  Top 0.152: J24.P$49 v6.83,22 | v31.3,2.2 24.2,9.3 16.9,9.3 16.2,10 16.2,21.3 16.02,21.3 15.79,21.53 13.32,21.53 v13.3,21.55 | S2.P$3 S2.P$6
  Bottom 0.152: v6.83,22 10.1,22 11.3,23.2 12.8,23.2 13.3,22.7 v13.3,21.55 | v31.3,2.2 31.4,2.1 S2.P$6
  other vias: 43.5,2.1
DRV_EN_DRV  (via drill 0.3)
  Top 0.152: U5.P$16 16.52,34 16.2,33.67 12.88,33.67 R8.2 11.25,34.25 v11.2,34.2 | S2.P$2 S2.P$5 40.43,2.1 v39.9,2.63 | v30.73,3.52 30.55,3.7 30.23,3.7 24.33,9.61 17.03,9.61 16.5,10.13 16.5,21.2 16.5,21.47 16.22,21.75 v16.22,23.42
  Bottom 0.152: v39.9,2.63 39.67,2.4 31.85,2.4 31.52,2.73 31.07,2.73 30.9,2.9 30.9,3.35 v30.73,3.52 | v16.22,23.42 13.01,23.42 12.93,23.5 11.17,23.5 9.97,22.3 8.1,22.3 6.83,23.57 6.83,23.72 6.46,24.09 5.25,24.09 5.02,23.87 4.58,23.87 4.07,24.38 4.07,26.42 4.38,26.73 4.58,26.73 11.2,33.35 v11.2,34.2
DRV_FAULT  (via drill 0.3)
  Top 0.152: U5.P$6 17.87,38.87 17.13,38.87 16.84,38.58 v16.7,38.58 | v10.31,28.17 10.31,27.44 9.85,26.98 9.85,26.34 9.59,26.08 9.59,20.39 9.4,20.2 J24.P$46
  Bottom 0.152: v16.7,38.58 16.7,38.51 16.23,38.04 16.23,37.72 16.02,37.51 15.9,37.51 15.23,36.84 15.23,36.52 10.59,31.88 10.59,28.3 10.46,28.17 v10.31,28.17
DRV_OCTW  (via drill 0.3)
  Top 0.152: U5.P$5 16.94,39.5 v16.78,39.33 | v9.76,27.64 9.76,27.32 9.54,27.11 9.54,26.47 9.28,26.2 9.28,21.58 9.1,21.4 J24.P$48
  Bottom 0.152: v16.78,39.33 16.55,39.11 16.48,39.11 16.17,38.8 16.17,38.41 15.92,38.17 15.92,37.97 14.93,36.97 14.93,36.65 10.28,32 10.28,28.7 10.09,28.7 9.76,28.37 v9.76,27.64
ENC_CSN  (via drill 0.3)
  Top 0.152: J2.5 13.5,5.7 9.7,9.5 v9.6,9.5 | v6.4,14.1 7.1,14.8 J24.P$37
  Bottom 0.152: v9.6,9.5 9.6,10.7 6.4,13.9 v6.4,14.1
ENC_MISO
  Top 0.152: J24.P$34 6.57,13 6,12.43 6,10.08 11.8,4.27 14.97,4.27 15.5,4.8 J2.3
ENC_MOSI
  Top 0.152: J24.P$33 6.9,12.4 6.7,12.2 6.7,11.07 J2.6
ENC_SCK
  Top 0.152: J24.P$36 9,14.2 9.9,13.3 9.9,10.4 14.5,5.8 J2.4
GND  (via drill 0.3, 0.35)  (16 unrouted)
  Top 0.203: 23.15,35.58 v23.01,35.72 | 23.15,38.18 v23.01,38.32
  other vias: 20.47,37.5 21.74,37.5 23.01,37.5 20.47,36.61 20.47,35.72 20.47,34.83 20.47,33.06 20.47,33.95 20.47,32.17 21.74,36.61 21.74,35.72 23.01,36.61 23.01,34.83 21.75,34.75 21.74,33.95 21.74,33.06 21.74,32.17 23.01,33.95 23.01,33.06 23.01,32.17 29.05,40.9 28.9,39.6 28.5,27 28.5,26 28.5,25 20.47,40.1 21.74,40.1 23.01,40.1 20.47,39.21 20.47,38.32 21.74,39.21 21.74,38.32 23.01,39.21 20.47,31.4 21.74,31.4 23.01,31.4 20.47,30.51 20.47,29.62 21.74,30.51 21.74,29.62 23.01,30.51 23.01,29.62 19.97,27.12 19.97,26.32 21.77,27.12 12.4,30.15 12.4,29.35 13.4,37.2 15.4,40.7 14.6,40.7 28.5,24 28.5,23 28.5,22 36.5,15.5 33.9,27.8 33.2,39 15.4,31.2 15.5,26.9 18.2,27.1 28.2,28.6 29.5,27 23.9,19.2 31.2,19.2 21.6,20.3 31.7,5.3 36.7,38.3 36.7,37.6 29.7,36.9 30.9,37.1 32.2,35.8 32.2,38 36,38.3 36,37.6 35.3,37.6 35.3,38.3 35.3,39 36,39 36.7,39 36.7,39.7 36,39.7 35.3,39.7 34.6,39.7 34.6,39 33.2,38 32.2,37.1 34.6,27.8 35.3,27.8 36,27.8 36.7,27.8 36.7,27.1 36,27.1 35.3,27.1 34.6,27.1 33.9,27.1 34.6,26.4 35.3,26.4 36,26.4 36.7,26.4 36.7,24.7 35,24.7 35.1,29.4 33.3,29.4 33.3,25.9 35.5,15.5 34.5,15.5 34,14.5 35,14.5 36,14.5 35.5,13.5 34.5,13.5 36.5,13.5 36,12.5 35,12.5 36.5,9 35.5,9 34.5,9 34,8 35,8 36,8 35.5,7 34.5,7 36.5,7 36,6 35,6 34,12.5 36.5,4.5 12.3,42.2 7.3,9.7 10.5,6.5 10.5,10.9 8.8,10.3 11.2,21.6 29,25.5 29,23.5 29,22.5 24.7,16.9 26.6,16.9 17.4,12.5 17.4,16.5 13.9,16.5 13.9,12.5 13.9,20.5 17.4,20.5 12,46 12.5,45.5 13,45 13.5,45.5 14,45 14,46 13,46 12,45 20,46 20.5,45.5 21,45 21.5,45.5 22,45 22,46 21,46 20,45 28,46 28.5,45.5 29,45 29.5,45.5 30,45 30,46 29,46 28,45 36,46 36.5,45.5 37,45 37.5,45.5 38,45 38,46 37,46 36,45 54.5,46 54.5,45 55.5,45 55.5,46 74.5,46 74.5,45 75.5,45 75.5,46 69.5,46 69.5,45 70.5,45 70.5,46 64.5,46 64.5,45 65.5,45 65.5,46 59.5,46 59.5,45 60.5,45 60.5,46 74.5,2 74.5,1 75.5,1 75.5,2 69.5,2 69.5,1 70.5,1 70.5,2 64.5,2 64.5,1 65.5,1 65.5,2 59.5,2 59.5,1 60.5,1 60.5,2 84,39.5 84,38.5 85,38.5 85,39.5 84,18.7 84,17.7 85,17.7 85,18.7 84,29.3 84,28.3 85,28.3 85,29.3 31.7,30.7 29.6,32.2 31.3,32 18.4,17.7 10.1,15.5 13,8.6 23.7,8.6 25,10 32.3,3.1 30,2.4 4.5,17.7 6.2,19.5 4.2,29.3 8.8,29.4 12.3,28 9.2,34.1 1,35.1 9.8,39.6
  pour Bottom (rank 6): -3,56.5 93,56.5 93,-5 -3,-5
  pour Top (rank 6): -5,58.5 95,58.5 95,-7 -5,-7
  pour Top (rank 3, no thermals): 47,16.2 33.5,16.2 33.5,-1 47,-1
  pour Top (rank 3, no thermals): 37.2,27.9 37.2,25.7 33.6,25.7 33.6,27.9
  pour Top (rank 3, no thermals): 33.6,40.4 37.2,40.4 37.2,38.2 33.6,38.2
  pour Route2 (rank 6): -4.5,58 94.5,58 94.5,-6.5 -4.5,-6.5
  pour Route15 (rank 6): -3.5,57 93.5,57 93.5,-5.5 -3.5,-5.5
I-V  (via drill 0.3, 0.35)
  Top 0.203: U5.P$25 16.76,29.5 v16.23,28.97 | v4.6,26.2 J24.P$5
  Bottom 0.203: v16.23,28.97 15.91,28.97 12.14,25.2 5.9,25.2 4.9,26.2 v4.6,26.2
I-W  (via drill 0.3, 0.35)
  Top 0.203: U5.P$26 v19.27,29 | v19.27,29 | J24.P$6 4.4,25.6 v4.6,25.4
  Bottom 0.203: v19.27,29 18.63,28.37 16.52,28.37 16.49,28.34 15.96,28.34 15.91,28.39 15.1,27.59 15.03,27.59 12.24,24.8 5.7,24.8 5.1,25.4 v4.6,25.4
M_GAIN  (via drill 0.3)
  Top 0.152: U5.P$10 16.78,37 v16.75,37.02 | v10.97,27.24 10.97,26.6 10.2,25.83 10.2,18.2 9.79,17.8 J24.P$42
  Bottom 0.152: v16.75,37.02 16.63,36.9 16.15,36.9 15.84,36.59 15.84,36.27 11.2,31.62 11.2,27.47 v10.97,27.24
M_PWM  (via drill 0.3)
  Top 0.152: U5.P$8 16.94,38 v16.76,37.82 | v10.38,26.76 10.38,26.44 9.89,25.95 9.89,19.79 9.7,19.6 J24.P$45
  Bottom 0.152: v16.76,37.82 16.14,37.2 16.02,37.2 15.54,36.71 15.54,36.39 10.89,31.75 10.89,28 10.38,27.49 v10.38,26.76
N$2  (via drill 0.3)  (1 unrouted)
  Top 0.203: 36.2,31.09 R18.2 36.15,31.05 44.66,31.05 Q2.P$4
  Bottom 0.203: Q2.P$4 37.5,32.59 37.5,39.1 46.14,39.1 v46.2,39.04
  other vias: 46.2,32.59
N$3  (via drill 0.3)
  Top 0.203: Q3.P$4 72.9,36.55 66.4,36.55 | 66.4,36.55 Q1.P$4 | v61.4,36.55 66.4,36.55 | R17.2 31.8,41.1 35.7,41.1 v36.1,41.5
  Bottom 0.203: v61.4,36.55 61.4,44.1 37.4,44.1 37.4,41.9 37.05,41.55 36.15,41.55 v36.1,41.5
N$4  (via drill 0.3)
  Top 0.203: Q5.P$4 72.9,22.5 66.4,22.5 | 66.4,22.5 v61.6,22.5 | Q7.P$4 66.4,22.5 | R24.2 36.36,29 v37.4,30.04
  Bottom 0.203: v61.6,22.5 61.4,22.7 61.4,31.3 37.4,31.3 v37.4,30.04
N$5  (via drill 0.3)
  Top 0.203: R31.2 36.25,17.3 | Q11.P$4 72.9,8.5 66.4,8.5 | 66.4,8.5 v61.4,8.5 | Q9.P$4 66.41,8.49 66.4,8.5
  Bottom 0.203: R31.2 37.15,16.4 61.4,16.4 v61.4,8.5
  other vias: 36.05,17.5
N$6  (via drill 0.3)
  Bottom 0.203: R32.2 37.4,10.95 | 37.4,10.95 46.05,10.95 Q12.P$4 | 37.4,10.95 37.5,10.85 37.5,4.5 46.1,4.5 Q10.P$4
  other vias: 35.05,10.95 46.2,11.1 46.2,4.59
N$7
  Top 0.203: U5.P$38 27.38,32.5 27.66,32.21 28.68,32.21 29.09,31.8 29.09,31.51 C30.1
N$8
  Top 0.203: U5.P$43 C29.1 | C29.1
N$9
  Top 0.203: U5.P$48 27.45,37.5 C28.1
N$10
  Top 0.203: U5.P$55 | U5.P$55 26.6,41 26.7,40.9 R11.2
N$11
  Top 0.203: U5.P$27 | U5.P$27 17,28.5 16.85,28.35 C20.2
N$13
  Top 0.203: U5.P$33 25.45,29.95 24.32,29.95 23.2,28.83 23.2,27.23 23.28,27.15 23.28,26.66 22.51,25.89 22.42,25.81 21.61,25.81 21.29,25.5 20.05,25.5 C26.1 19.1,24.45 R12.2
N$14
  Top 0.203: U5.P$32 25.44,29.45 24.39,29.45 23.61,28.66 23.61,27.4 23.69,27.32 23.69,26.41 22.58,25.41 21.77,25.41 20.97,24.6 C26.2 20.95,23.4 R13.2
N$15
  Top 0.203: U5.P$31 25.44,28.95 24.47,28.95 24.01,28.49 24.01,27.57 24.09,27.49 24.09,26.24 C27.1 22.35,23.4 R14.2
N$16
  Top 0.203: U5.P$30 24.6,28.5 24.42,28.32 24.42,27.73 24.5,27.66 24.5,24.85 C27.2 24.25,23.4 R15.2
N$18
  Top 0.203: U5.P$13 16.73,35.5 16.47,35.76 15.64,35.76 C16.2 15.1,36.3 | 15.1,36.3 15,36.4 C15.2 | 15.1,36.3
N$19
  Top 0.203: U5.P$49 26.5,38 27.2,38.7 27.2,39.5 C25.1
N$20
  Top 0.203: U5.P$11 18.84,36.5 19.08,36.27 19.08,30.73 18.84,30.5 U5.P$23 15.9,30.5 14.9,29.5 C17.2
N$21
  Top 0.152: U5.P$7 | U5.P$7 18.13,38.63 18.87,38.63 19,38.77 19,41.73 18.87,41.87 18.81,41.87 13.92,41.87 R10.1
N$24  (via drill 0.3)
  Top 0.203: R25.2 36.6,19.2 37.2,18.59 Q8.P$4
  Bottom 0.203: Q8.P$4 37.7,18.6 37.7,25.1 37.7,25.09 Q6.P$4
  other vias: 46.2,18.59 46.2,25.09
N$25
  Top 0.152: U5.P$9 18.13,37.63 18.87,37.63 19,37.77 19,38.34 19.31,38.64 19.31,41.86 19,42.17 13.57,42.17 12.93,41.53 12.08,41.53 R9.1
PHASE-U  (via drill 0.3, 0.35)
  Top 0.203: U5.P$46 26.34,36.5 26.35,36.51 28.31,36.51 29.12,37.32 29.12,37.57 C28.2 31.1,38 33.8,40.7 36.6,40.7 37.5,41.6 37.5,43.4 37.7,43.6 48.1,43.6 49.95,41.75 Q4.P$5 | v19.2,19.1 18.05,20.25 18.05,21.2 17.45,21.81 R20.2
  Bottom 0.203: 47.9,32.1 47.46,31.66 37.25,31.66 37.04,31.45 37.04,30.47 36.84,30.27 36.84,29.81 37.34,29.31 37.34,19.14 36.86,18.66 36.66,18.66 36.41,18.41 35.67,18.41 35.52,18.26 20.04,18.26 v19.2,19.1
  other vias: 52,43 52,42 52,41 52,40 52,39 51,39.5 51,40.5 51,41.5 51,42.5 50,43 50,42 50,41 50,40 50,39 49,39.5 49,40.5 49,41.5 49,42.5 52,36.5 52,35.5 52,34.5 52,33.5 52,32.5 51,33 51,34 51,35 51,36 50,36.5 50,35.5 50,34.5 50,33.5 50,32.5 49,33 49,34 49,35 49,36 64,32.5 64,33.5 65,34.5 65,33.5 65,32.5 60,43 51,37 49,37 49,38.5 51,38.5 51,43.5 49,43.5 51,32 49,32 48,43 48,42 48,41 48,40 48,39 48,36.5 48,35.5 48,34.5 48,33.5 48,32.5 60,32.5
  pour Top (rank 4, no thermals): 61.5,43.7 47,43.7 47,31.5 88,31.5 88,36.5 61.5,36.5
  pour Bottom (rank 3, no thermals): 61.39,44.1 37.5,44.1 37.5,31.5 66,31.5 66,36 61.5,36
PHASE-V  (via drill 0.3, 0.35)
  Top 0.203: U5.P$41 27.14,34 27.2,33.94 28.16,33.94 28.51,33.59 31.84,33.59 31.85,33.6 | C29.2 30.79,35 31.85,33.94 31.85,33.6 | 31.85,33.6 31.85,33.38 33,32.23 33,30.79 33.7,30.1 36.51,30.1 37,30.59 44.7,30.59 45.15,31.05 47.45,31.05 v48,30.5 | v19.21,18.31 19.01,18.5 R22.2
  Bottom 0.203: 48,17.5 47.26,16.76 37.3,16.76 36.61,17.45 36.61,17.73 36.28,18.06 35.82,18.06 35.66,17.9 32.9,17.9 19.61,17.9 v19.21,18.31
  other vias: 52,29 52,28 52,27 52,26 52,25 51,25.5 51,26.5 51,27.5 51,28.5 50,29 50,28 50,27 50,26 50,25 49,25.5 49,26.5 49,27.5 49,28.5 52,22.5 52,21.5 52,20.5 52,19.5 52,18.5 51,19 51,20 51,21 51,22 50,22.5 50,21.5 50,20.5 50,19.5 50,18.5 49,19 49,20 49,21 49,22 64,18.5 64,19.5 65,20.5 65,19.5 65,18.5 51,29.5 49,29.5 51,24.5 49,24.5 51,23 49,23 51,18 49,18 48,29 48,28 48,27 48,26 48,25 48,22.5 48,21.5 48,20.5 48,19.5 48,18.5 60,30 53.5,17.5
  pour Top (rank 4, no thermals): 47,31.2 47,16.5 61.5,16.5 61.5,17.5 88,17.5 88,24.3 79.3,24.3 79.3,22.3 61.5,22.3 61.5,31.2
  pour Bottom (rank 3, no thermals): 66,17.5 61.5,17.5 61.5,16.5 37.5,16.5 37.5,31 61.5,31 61.5,22 66,22
PHASE-W  (via drill 0.3, 0.35)
  Top 0.203: U5.P$36 27.3,31.5 27.35,31.45 27.55,31.45 C30.2 28.36,30.64 28.36,30.43 28.74,30.04 30.95,30.04 31.58,29.42 31.58,25.04 31.98,24.64 31.98,22.08 31.58,21.68 31.58,20.92 32.69,19.81 32.69,19.41 33.19,18.91 33.19,18.35 33.55,17.99 33.55,16.8 33.8,16.54 35.1,16.54 | 35.1,16.54 47,16.54 47.5,16.04 47.5,15.7 | v35.1,17.1 35.1,16.54 | R27.2 17.5,14.5 17.5,15.5 17.65,15.65 17.91,15.65 18.05,15.79 18.05,16.05 v19.3,17.3
  Bottom 0.203: v35.1,17.1 34.66,17.54 19.54,17.54 v19.3,17.3
  other vias: 52,15 52,14 52,13 52,12 52,11 51,11.5 51,12.5 51,13.5 51,14.5 50,15 50,14 50,13 50,12 50,11 49,11.5 49,12.5 49,13.5 49,14.5 52,8.5 52,7.5 52,6.5 52,5.5 52,4.5 51,5 51,6 51,7 51,8 50,8.5 50,7.5 50,6.5 50,5.5 50,4.5 49,5 49,6 49,7 49,8 60.5,6.5 60.5,7.5 60.5,5.5 60.5,4.5 60.5,3.5 51,15.5 49,15.5 51,10.5 49,10.5 51,9 49,9 51,4 49,4 48,15 48,14 48,13 48,12 48,11 48,8.5 48,7.5 48,6.5 48,5.5 48,4.5 59.5,5 60.5,15.5 48,1
  pour Top (rank 4, no thermals): 61.5,16.2 61.5,8.3 79.3,8.3 79.3,13 89,13 89,-1 47,-1 47,16.2
  pour Bottom (rank 3): 61.5,16.2 37.5,16.2 37.5,-0.5 61.5,-0.5
PWMHIU
  Top 0.152: U5.P$17 16.45,33.5 16.32,33.37 9.21,33.37 5.58,29.73 5.58,27.55 6.21,26.92 6.21,26.75 6.51,26.45 6.51,26.28 6.82,25.97 6.82,25.8 7.12,25.5 7.12,25.33 7.45,25 J24.P$54
PWMHIV
  Top 0.152: U5.P$19 16.47,32.5 16.21,32.76 9.46,32.76 6.19,29.48 6.19,27.8 6.82,27.17 6.82,27 7.12,26.7 7.12,26.53 7.25,26.4 8,26.4 J24.P$56
PWMHIW
  Top 0.152: U5.P$21 16.6,31.5 15.95,32.15 9.72,32.15 6.79,29.23 6.79,28.06 7.25,27.6 8,27.6 J24.P$58
PWMLOU
  Top 0.152: U5.P$18 16.4,33 16.34,33.06 13.2,33.06 13.15,33.06 9.34,33.06 5.88,29.61 5.88,27.68 6.51,27.05 6.51,26.88 6.82,26.57 6.82,26.4 7.12,26.1 7.12,25.93 7.25,25.8 8,25.8 J24.P$55
PWMLOV
  Top 0.152: U5.P$20 16.54,32 16.09,32.45 12.9,32.45 9.59,32.45 6.49,29.35 6.49,27.93 7.12,27.3 7.12,27.13 7.45,26.8 J24.P$57
PWMLOW
  Top 0.152: U5.P$22 16.67,31 15.83,31.84 9.84,31.84 7.1,29.1 7.1,28.2 7.3,28 J24.P$59
SHNT-U-HI  (via drill 0.3)
  Top 0.203: R19.SA v34.1,36 | v29.8,27.9 30.16,27.55 30.16,24.45 30.55,24.05 30.55,23.6 v30.35,23.4
  Bottom 0.203: v34.1,36 32.9,34.8 30.46,34.8 30.07,34.41 30.07,33.93 30.6,33.4 30.6,28.7 v29.8,27.9 | v30.35,23.4 30.5,23.25 30.5,23.18 30.16,22.84 30.16,22.37 30.36,22.17 30.36,21.42 30.2,21.27 25.24,21.27 25.11,21.39 25.11,21.73 24.58,22.26 20.01,22.26 R12.1
  other vias: 19.1,21.35
SHNT-U-LO  (via drill 0.3)
  Top 0.203: R19.SB v34.1,37.3 | v29.77,28.66 29.97,28.46 30.03,28.46 30.51,27.98 30.51,24.6 30.9,24.2 30.9,22.8 v30.71,22.6
  Bottom 0.203: v34.1,37.3 33.5,36.7 33.5,35.9 32.75,35.16 30.31,35.16 29.71,34.56 29.71,33.78 30.24,33.25 30.24,28.85 30.05,28.66 v29.77,28.66 | v30.71,22.6 30.71,21.01 30.61,20.91 25.09,20.91 24.76,21.24 24.76,21.58 24.43,21.91 21.36,21.91 R13.1
  other vias: 20.8,21.35
SHNT-V-HI  (via drill 0.3)
  Top 0.203: R26.SA v34.1,23.2
  Bottom 0.203: v34.1,23.2 32.76,21.86 32.26,21.86 31.93,21.53 31.93,21.03 31.1,20.2 22.9,20.2 22.5,20.6 R14.1
  other vias: 22.5,21.35
SHNT-V-LO  (via drill 0.3)  (1 unrouted)
  Top 0.203: R26.SB v34.1,24.7
  Bottom 0.203: v34.1,24.7 33.5,24.1 33.5,23.1 32.61,22.21 32.11,22.21 31.58,21.68 31.58,21.18 30.95,20.56 24.7,20.56 24.2,21.06 v24.2,21.35
SL-U  (via drill 0.3)
  Top 0.203: U5.P$44 25.55,35.56 26.48,35.56 26.66,35.74 30.55,35.74 32.41,33.89 v32.41,33.61
  Bottom 0.203: v32.41,33.61 33.79,33.61 v34.2,33.2
  pour Top (rank 3, no thermals): 47,31.5 47,43.7 37.5,43.7 37.5,36.5 34.5,36.5 34.5,34.5 33.5,34.5 33.5,31.5
SL-V  (via drill 0.3)
  Top 0.203: U5.P$39 27.95,33 28.17,32.77 31.45,32.77 32.29,31.93 32.29,25.33 32.69,24.93 32.69,21.6 32.49,21.4 v32.49,21.3
  Bottom 0.203: 32.59,21.2 v32.49,21.3 32.99,20.8 v33.9,20.8
  pour Top (rank 3, no thermals): 47,31.2 37.5,31.2 37.5,24 34.5,24 34.5,22 33.5,22 33.5,16.5 47,16.5
SL-W  (1 unrouted)
  Top 0.203: U5.P$34 25.55,30.45 | U5.P$34 | U5.P$34 26.76,30.5 27.17,30.09 27.69,30.09 28.45,29.33 30.66,29.33 30.87,29.12 30.87,24.74 31.27,24.34 31.27,22.37 30.87,21.97 30.87,20.63 31.98,19.52 31.98,19.11 32.48,18.61 32.48,18.05 32.74,17.79 32.74,11.85 32.55,11.65 32.55,10.24 32.7,10.1 32.96,10.1 33.16,9.9
V-U  (via drill 0.3)
  Top 0.152: R21.2 R20.1 D4.1 12.2,24.15 C31.1 13.69,26.14 14.1,26.14 v14.23,26.01 | J24.P$8 v4.8,24.4
  Top 0.203: 12.05,24.35 C31.1
  Bottom 0.152: v4.8,24.4 12.36,24.4 14.1,26.14 v14.23,26.01
V-V  (via drill 0.3)
  Top 0.152: R23.2 R22.1 D5.1 12.2,20.15 C33.1 v11.5,20.5 | v6.3,23.5 6,23.8 J24.P$9
  Bottom 0.152: v11.5,20.5 7.2,20.5 6.3,21.4 v6.3,23.5
V-VCC  (via drill 0.3)
  Top 0.152: R30.2 R29.1 D7.1 12.2,12.15 C38.1 v10.7,12.5 | v4.4,22 J24.P$12
  Bottom 0.152: v10.7,12.5 4.4,18.8 v4.4,22
V-W  (via drill 0.3)
  Top 0.152: R28.2 R27.1 D6.1 12.2,16.15 C37.1 v11.4,16.5 | v5.4,22.6 J24.P$11
  Bottom 0.152: v11.4,16.5 8.1,16.5 5.4,19.2 v5.4,22.6
VCC  (via drill 0.3, 0.35)  (4 unrouted)
  Top 0.152: R29.2 18.03,11.08 18.03,14.8 19.53,16.3 25.1,16.3 25.9,17.1 C35.1
  Top 0.203: 80.5,17.1 v80.5,16.5
  Top 1.27: C7.1 80.5,17.1
  other vias: 62.5,27.5 63.5,27.5 64.5,27.5 65.5,27.5 66.5,27.5 66,26.5 65,26.5 64,26.5 63,26.5 62.5,25.5 63.5,25.5 64.5,25.5 65.5,25.5 66.5,25.5 66,24.5 65,24.5 64,24.5 63,24.5 62.5,13.5 63.5,13.5 64.5,13.5 65.5,13.5 66.5,13.5 66,12.5 65,12.5 64,12.5 63,12.5 62.5,11.5 63.5,11.5 64.5,11.5 65.5,11.5 66.5,11.5 66,10.5 65,10.5 64,10.5 63,10.5 69,13.5 70,13.5 71,13.5 72,13.5 73,13.5 72.5,12.5 71.5,12.5 70.5,12.5 69.5,12.5 69,11.5 70,11.5 71,11.5 72,11.5 73,11.5 72.5,10.5 71.5,10.5 70.5,10.5 69.5,10.5 69,27.5 70,27.5 71,27.5 72,27.5 73,27.5 72.5,26.5 71.5,26.5 70.5,26.5 69.5,26.5 69,25.5 70,25.5 71,25.5 72,25.5 73,25.5 72.5,24.5 71.5,24.5 70.5,24.5 69.5,24.5 62.5,41.5 63.5,41.5 64.5,41.5 65.5,41.5 66.5,41.5 66,40.5 65,40.5 64,40.5 63,40.5 62.5,39.5 63.5,39.5 64.5,39.5 65.5,39.5 66.5,39.5 66,38.5 65,38.5 64,38.5 63,38.5 69,41.5 70,41.5 71,41.5 72,41.5 73,41.5 72.5,40.5 71.5,40.5 70.5,40.5 69.5,40.5 69,39.5 70,39.5 71,39.5 72,39.5 73,39.5 72.5,38.5 71.5,38.5 70.5,38.5 69.5,38.5 62.5,30.5 63.5,30.5 64.5,30.5 65.5,30.5 66.5,30.5 69,30.5 70,30.5 71,30.5 72,30.5 73,30.5 62.5,16.5 63.5,16.5 64.5,16.5 65.5,16.5 66.5,16.5 69,16.5 70,16.5 71,16.5 72,16.5 73,16.5 62.5,47.5 63.5,47.5 64.5,47.5 65.5,47.5 66.5,47.5 69,47.5 70,47.5 71,47.5 72,47.5 73,47.5 78.5,25.5 79.5,26.5 79.5,15.5 67,10.5 67,12.5 62,12.5 62,10.5 68.5,12.5 68.5,10.5 73.5,10.5 73.5,12.5 67,26.5 67,24.5 62,24.5 62,26.5 68.5,26.5 68.5,24.5 73.5,24.5 73.5,26.5 67,40.5 67,38.5 62,40.5 62,38.5 68.5,38.5 68.5,40.5 73.5,40.5 73.5,38.5 62.5,37.5 63.5,37.5 64.5,37.5 65.5,37.5 66.5,37.5 69,37.5 70,37.5 71,37.5 72,37.5 73,37.5 62.5,23.5 63.5,23.5 64.5,23.5 65.5,23.5 66.5,23.5 69,23.5 70,23.5 71,23.5 72,23.5 73,23.5 62.5,9.5 63.5,9.5 64.5,9.5 65.5,9.5 66.5,9.5 69,9.5 70,9.5 71,9.5 72,9.5 73,9.5 26,26 25.5,25.5 26,25 25.5,24.5 26,24 25.5,23.5 26,23 25.5,22.5 26,22 77.5,2 77.5,1 78.5,1 78.5,2 72.5,2 72.5,1 73.5,1 73.5,2 67.5,2 67.5,1 68.5,1 68.5,2 62.5,2 62.5,1 63.5,1 63.5,2
  pour Top (rank 3, no thermals): 24.7,28.2 26.75,28.2 26.75,18.5 24.8,18.5 24.8,27.7 24.7,27.8
  pour Top (rank 5, no thermals): 92,51.5 61.5,51.5 61.5,-3.5 92,-3.5
  pour Bottom (rank 4, no thermals): 61.5,52 90,52 90,-4 61.5,-4
  pour Bottom: -0.5,36 9,36 9,40 12,43 31,43 36,43 37,44 62.5,44 62.5,53 -1,53 -1,36.5
  pour Top (no thermals): 9,36 9,40 12,43 36,43 37,44 63,44 63,53.5 -1.5,53.5 -1.5,36.5 -1,36
  pour Route15: -2,36 9,36 9,40 12,43 23,43 25,41 25,18.8 27.5,18.8 27.5,42 28.5,43 36,43 37,44 61.5,44 61.5,-4.5 92.5,-4.5 92.5,52.5 -2,52.5

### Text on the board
tPlace: VCC | U | V | W | atkbldcdriver v0.62 | < no - go > | GND | SPI
bPlace: He said, 'no, I mean God like physics'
